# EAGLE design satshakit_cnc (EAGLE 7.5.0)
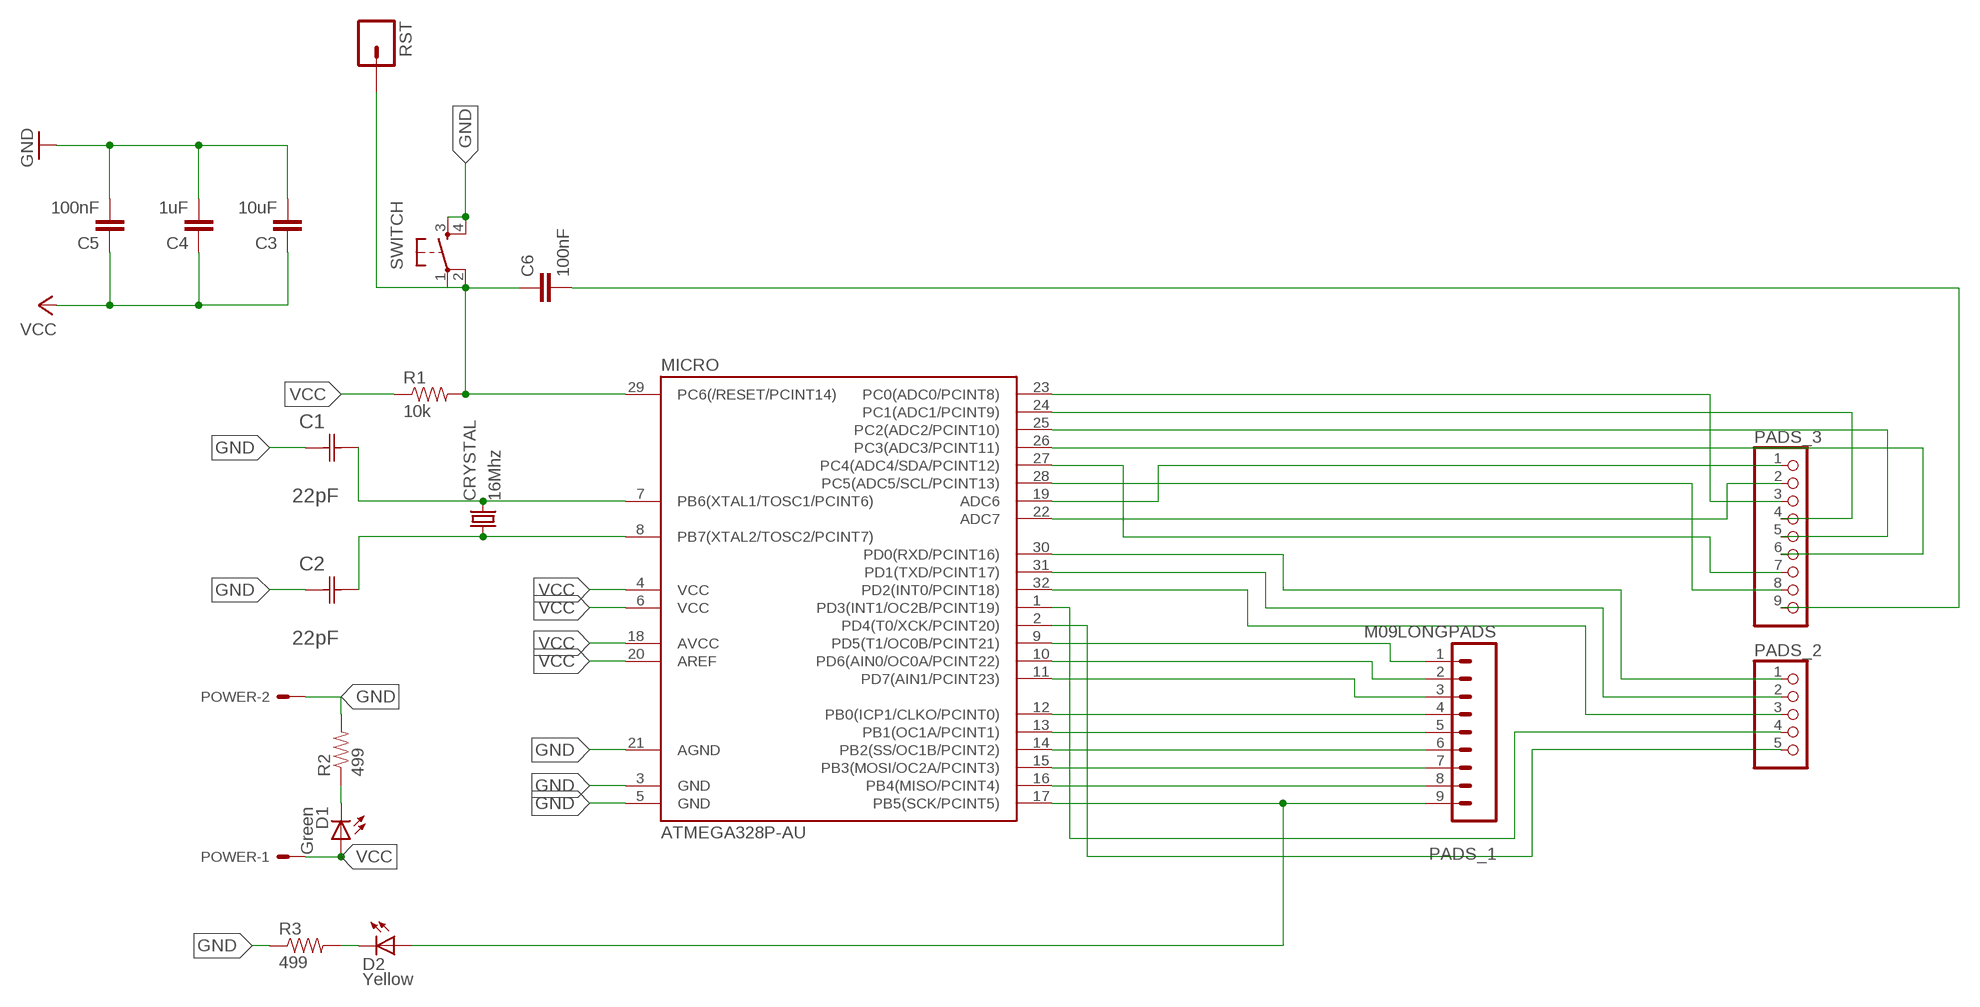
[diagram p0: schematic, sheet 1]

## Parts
C1  22pF  0612ZC225MAT2A  [CAPC3216X178N]
C2  22pF  0612ZC225MAT2A  [CAPC3216X178N]
C3  10uF  CAP1206  [1206]
C4  1uF  CAP1206  [1206]
C5  100nF  CAP1206  [1206]
C6  100nF  CAP1206  [1206]
CRYSTAL  16Mhz  CSM-7X-DU  [CSM-7X-DU]
D1  Green  LED1206  [1206]
D2  Yellow  LED1206  [1206]
MICRO  ATMEGA328P-AU  ATMEGA48/88/168-AU  [TQFP32-08]
PADS_1  M09LONGPADS  [1X09_LONGPADS]
PADS_2  PINHD-1X5  [1X05]
PADS_3  PINHD-1X9  [1X09]
POWER  22-23-2021  [22-23-2021]
R1  10k  RESISTOR1206  [1206]
R2  499  RESISTOR1206  [1206]
R3  499  RESISTOR1206  [1206]
RST  M01PTH  [1X01]
SWITCH  6MM_SWITCH6MM_SWITCH  [6MM_SWITCH]

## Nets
GND: C1.1(C1) C2.1(C1) C3.2 C4.2 C5.2 MICRO.3(GND) MICRO.5(GND) MICRO.21(AGND) POWER.2 R2.2 R3.1 SWITCH.3(S) SWITCH.4(S1)
N$1: MICRO.9(PD5(T1/OC0B/PCINT21)) PADS_1.1
N$2: C1.2(C2) CRYSTAL.2 MICRO.7(PB6(XTAL1/TOSC1/PCINT6))
N$3: C6.2 PADS_3.9
N$4: MICRO.10(PD6(AIN0/OC0A/PCINT22)) PADS_1.2
N$5: MICRO.11(PD7(AIN1/PCINT23)) PADS_1.3
N$6: MICRO.12(PB0(ICP1/CLKO/PCINT0)) PADS_1.4
N$7: MICRO.13(PB1(OC1A/PCINT1)) PADS_1.5
N$8: MICRO.14(PB2(SS/OC1B/PCINT2)) PADS_1.6
N$9: C2.2(C2) CRYSTAL.1 MICRO.8(PB7(XTAL2/TOSC2/PCINT7))
N$10: MICRO.15(PB3(MOSI/OC2A/PCINT3)) PADS_1.7
N$11: MICRO.16(PB4(MISO/PCINT4)) PADS_1.8
N$12: D2.1(A) MICRO.17(PB5(SCK/PCINT5)) PADS_1.9
N$13: MICRO.19(ADC6) PADS_3.1
N$14: MICRO.22(ADC7) PADS_3.2
N$15: MICRO.23(PC0(ADC0/PCINT8)) PADS_3.3
N$16: MICRO.24(PC1(ADC1/PCINT9)) PADS_3.4
N$17: MICRO.25(PC2(ADC2/PCINT10)) PADS_3.5
N$18: MICRO.26(PC3(ADC3/PCINT11)) PADS_3.6
N$19: MICRO.27(PC4(ADC4/SDA/PCINT12)) PADS_3.7
N$20: MICRO.30(PD0(RXD/PCINT16)) PADS_2.1
N$21: MICRO.31(PD1(TXD/PCINT17)) PADS_2.2
N$22: MICRO.32(PD2(INT0/PCINT18)) PADS_2.3
N$23: MICRO.1(PD3(INT1/OC2B/PCINT19)) PADS_2.4
N$24: MICRO.2(PD4(T0/XCK/PCINT20)) PADS_2.5
N$25: MICRO.28(PC5(ADC5/SCL/PCINT13)) PADS_3.8
N$26: D1.2(C) R2.1
N$27: D2.2(C) R3.2
N$28: C6.1 MICRO.29(PC6(/RESET/PCINT14)) R1.2 RST.1 SWITCH.1(P) SWITCH.2(P1)
VCC: C3.1 C4.1 C5.1 D1.1(A) MICRO.4(VCC) MICRO.6(VCC) MICRO.18(AVCC) MICRO.20(AREF) POWER.1 R1.1

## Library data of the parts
C1 C2 = AVX_By_element14_Batch_1:0612ZC225MAT2A: Capacitor 1206; MPN: 0612ZC225MAT2A; OC_FARNELL: -; OC_NEWARK: 12N3209; SUPPLIER: AVX; TOLERANCE: ±20%; VALUE: 2.2µF; VOLTAGERATING: 10V
C3-C6 = 01_SparkFun:CAP: Capacitor
CRYSTAL = 01_FAB_Hello:CSM-7X-DU: SMD CRYSTAL; OC_FARNELL: unknown; OC_NEWARK: unknown
D1 D2 = 01_FAB_Hello:LED
MICRO = atmega8:ATMEGA48/88/168
PADS_1 = 01_SparkFun:M09: Header 9 Standard 9-pin 0.1" header. Use with straight break away headers (SKU : PRT-00116), right angle break away headers (PRT-00553), swiss pins (PRT-00743), machine pins (PRT-00117), and female headers (PRT-00115).
PADS_2 = pinhead:PINHD-1X5: PIN HEADER
PADS_3 = pinhead:PINHD-1X9: PIN HEADER
POWER = con-molex:22-23-2021: .100" (2.54mm) Center Header - 2 Pin; MF: MOLEX; MPN: 22-23-2021; OC_FARNELL: 1462926; OC_NEWARK: 25C3832
R1-R3 = 01_SparkFun:RESISTOR: Resistor
RST = 01_SparkFun:M01: Header 1
SWITCH = 01_FAB_Hello:6MM_SWITCH: OMRON SWITCH

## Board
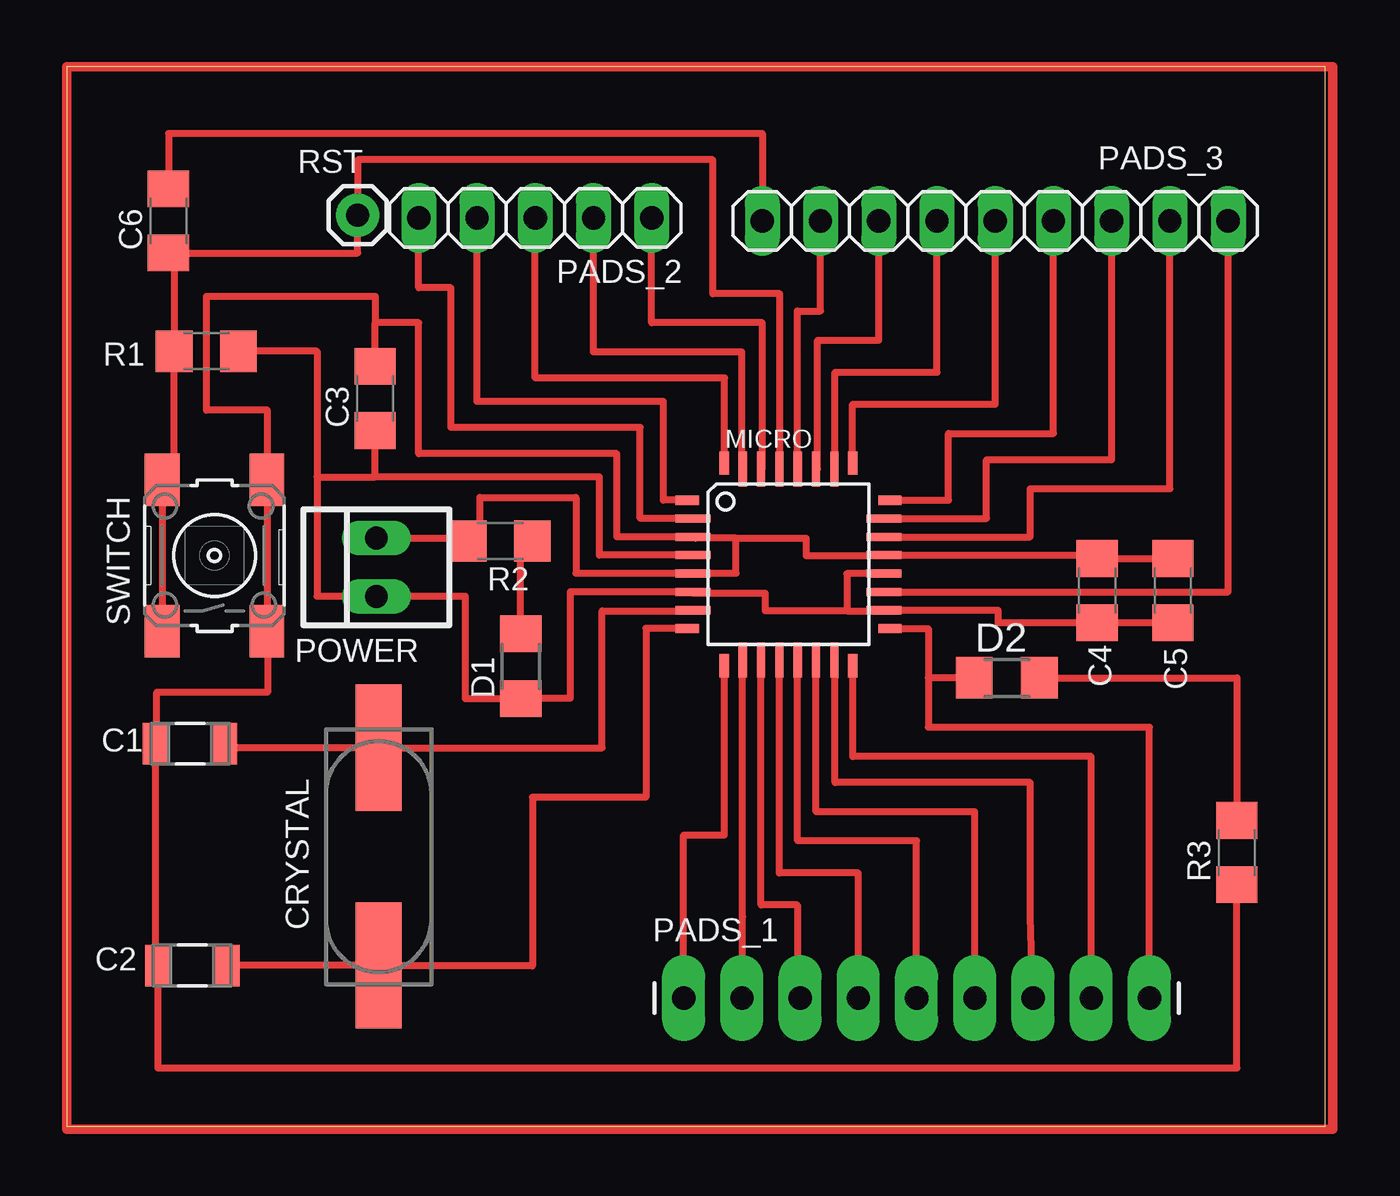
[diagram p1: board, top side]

Size 54.91 x 46.22 mm. Coordinates in mm from the lower left corner, seen from the top.
Outline: 0,0 54.91,0 54.91,46.22 0,46.22 0,0
Copper layers (1*16): Top 0.035mm / dielectric 1.5mm / Bottom 0.035mm
Design rules "default": minimum track width 10mil, minimum drill 24mil, track to track 8mil, track to pad 8mil, pad to pad 8mil, via to via 8mil, smd to smd 8mil, copper to edge 40mil, drill to drill 8mil, minimum pad ring 10mil, minimum via ring 8mil, stop-mask expansion 4mil, vias tented up to drill 0mil, thermal gap 10mil

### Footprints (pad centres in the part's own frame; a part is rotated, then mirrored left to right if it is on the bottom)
CAPC3216X178N = smd 1.118 x 1.803: 1 -1.499,0; 2 1.499,0
1206 = smd 1.6 x 1.8: 1 -1.4,0; 2 1.4,0
CSM-7X-DU = smd 5.5 x 2: 1 -4.75,0; 2 4.75,0
1206' = smd 1.6 x 1.803: 1 -1.422,0; 2 1.422,0
TQFP32-08 = smd 1.016 x 0.406: 1 -4.42,2.8; 8 -4.42,-2.8; 17 4.42,-2.8; 24 4.42,2.8 | smd 1.524 x 0.356: 2 -4.166,2; 3 -4.166,1.2; 4 -4.166,0.4; 5 -4.166,-0.4; 6 -4.166,-1.2; 7 -4.166,-2; 18 4.166,-2; 19 4.166,-1.2; 20 4.166,-0.4; 21 4.166,0.4; 22 4.166,1.2; 23 4.166,2 | smd 0.406 x 1.016: 9 -2.8,-4.42; 16 2.8,-4.42; 25 2.8,4.42; 32 -2.8,4.42 | smd 0.356 x 1.524: 10 -2,-4.166; 11 -1.2,-4.166; 12 -0.4,-4.166; 13 0.4,-4.166; 14 1.2,-4.166; 15 2,-4.166; 26 2,4.166; 27 1.2,4.166; 28 0.4,4.166; 29 -0.4,4.166; 30 -1.2,4.166; 31 -2,4.166
1X09_LONGPADS = drill 1.016 pad 1.88 long: 1 0,0; 2 2.54,0; 3 5.08,0; 4 7.62,0; 5 10.16,0; 6 12.7,0; 7 15.24,0; 8 17.78,0; 9 20.32,0
1X05 = drill 1.016 long: 1 -5.08,0; 2 -2.54,0; 3 0,0; 4 2.54,0; 5 5.08,0
1X09 = drill 1.016 long: 1 -10.16,0; 2 -7.62,0; 3 -5.08,0; 4 -2.54,0; 5 0,0; 6 2.54,0; 7 5.08,0; 8 7.62,0; 9 10.16,0
22-23-2021 = drill 1 long: 1 -1.27,0; 2 1.27,0
1X01 = drill 1.016 pad 1.88: 1 0,0
6MM_SWITCH = smd 2.286 x 1.524: 1 -3.302,2.286; 2 3.302,2.286; 3 -3.302,-2.286; 4 3.302,-2.286

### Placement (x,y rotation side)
C1  5.38,16.69 0 top
C2  5.49,7.01 0 top
C3  13.46,31.75 90 top
C4  44.96,23.37 90 top
C5  48.26,23.37 90 top
C6  4.45,39.5 90 top
CRYSTAL  13.61,11.76 90 top
D1  Green  [1206']  19.81,20.07 90 top
D2  Yellow  [1206']  41.02,19.56 0 top
MICRO  31.5,24.51 0 top
PADS_1  26.92,5.59 0 top
PADS_2  20.45,39.62 180 top
PADS_3  40.51,39.5 180 top
POWER  13.51,24.38 90 top
R1  6.1,33.81 180 top
R2  18.92,25.53 180 top
R3  51.05,11.94 90 top
RST  12.7,39.75 0 top
SWITCH  6.45,24.89 90 top

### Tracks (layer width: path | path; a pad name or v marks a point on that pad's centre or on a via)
GND
  Top 0.254: 27.36,25.68 MICRO.3 27.46,25.65 | 27.94,24.13 28.19,24.13 | 35.66,24.89 MICRO.21
  Top 0.305: MICRO.5 | MICRO.21 44.96,24.91 C4.2 C5.2 | C1.1 3.89,7.01 C2.1 3.99,2.54 51.05,2.54 R3.1 | C1.1 3.81,16.69 | 27.33,24.13 22.23,24.13 22.23,27.43 18.03,27.43 18.03,25.4 R2.2 18.03,25.65 POWER.2 | 27.33,24.13 MICRO.5 | C1.1 3.94,16.69 3.94,18.92 8.76,18.92 8.76,21.59 | 27.94,24.13 MICRO.5 | MICRO.3 24,25.71 24,29.34 15.37,29.34 15.37,35.05 13.46,35.05 | C3.2 13.46,35.05 | SWITCH.3 8.76,21.59 | 8.76,21.59 8.76,27.56 8.74,27.56 SWITCH.4 8.76,28.19 8.76,31.24 6.1,31.24 6.1,36.2 13.46,36.2 13.46,35.05 | 27.33,24.13 29.21,24.13 29.21,25.65 | 29.21,25.65 27.46,25.65 | 29.21,25.65 32.26,25.65 32.26,24.89 35.66,24.89
N$1
  Top 0.305: PADS_1.1 26.92,12.7 28.7,12.7 MICRO.9
N$2
  Top 0.305: 6.88,16.51 C1.2 6.88,16.51 | MICRO.7 27.33,22.48 23.37,22.48 23.37,16.51 CRYSTAL.2 6.88,16.51
N$3
  Top 0.305: PADS_3.9 30.35,43.31 4.45,43.31 C6.2
N$4
  Top 0.305: PADS_1.2 29.5,9.14 MICRO.10
N$5
  Top 0.305: MICRO.11 30.3,9.65 31.88,9.65 31.88,6.22 32,6.22 PADS_1.3
N$6
  Top 0.305: 31.11,20.35 MICRO.12 31.1,11.05 34.54,11.05 PADS_1.4
N$7
  Top 0.305: PADS_1.5 37.08,12.45 31.9,12.45 MICRO.13
N$8
  Top 0.305: PADS_1.6 39.62,13.72 32.7,13.72 MICRO.14
N$9
  Top 0.305: 6.99,6.99 C2.2 | MICRO.8 25.27,21.72 25.27,14.35 20.32,14.35 20.32,6.99 13.61,6.99 CRYSTAL.1 C2.2 | C2.2
N$10
  Top 0.305: PADS_1.7 42.04,9.14 42.04,14.99 33.53,14.99 33.53,19.56 MICRO.15
N$11
  Top 0.305: MICRO.16 34.3,16.13 44.7,16.13 PADS_1.8
N$12
  Top 0.305: PADS_1.9 47.24,17.4 37.59,17.4 37.59,19.56 | D2.1 37.59,19.56 | MICRO.17 37.59,21.71 37.59,19.56
N$13
  Top 0.305: MICRO.19 50.67,23.31 PADS_3.1
N$14
  Top 0.305: MICRO.22 42.04,25.71 42.04,27.81 48.13,27.81 PADS_3.2
N$15
  Top 0.305: MICRO.23 40.13,26.51 40.13,29.08 45.59,29.08 PADS_3.3
N$16
  Top 0.305: MICRO.24 38.48,27.31 38.48,30.23 43.05,30.23 PADS_3.4
N$17
  Top 0.305: MICRO.25 34.29,31.5 40.51,31.5 PADS_3.5
N$18
  Top 0.305: MICRO.26 33.53,28.68 33.53,32.89 37.97,32.89 PADS_3.6
N$19
  Top 0.305: MICRO.27 32.77,28.68 32.77,34.29 35.43,34.29 PADS_3.7
N$20
  Top 0.305: MICRO.30 30.35,28.68 30.35,35.05 25.53,35.05 PADS_2.1
N$21
  Top 0.305: MICRO.31 29.46,28.68 29.46,33.78 22.99,33.78 PADS_2.2
N$22
  Top 0.305: MICRO.32 28.7,32.64 20.45,32.64 PADS_2.3
N$23
  Top 0.305: MICRO.1 26.04,27.31 26.04,31.62 17.91,31.62 PADS_2.4
N$24
  Top 0.305: MICRO.2 25.02,26.51 25.02,30.48 16.76,30.48 16.76,36.58 15.37,36.58 PADS_2.5
N$25
  Top 0.305: MICRO.28 31.88,28.68 31.88,35.56 32.89,35.56 PADS_3.8
N$26
  Top 0.305: 20.7,25.27 R2.1 20.32,25.15 19.81,25.15 D1.2
N$27
  Top 0.305: D2.2 51.05,19.56 R3.2
N$28
  Top 0.305: MICRO.29 31.11,28.68 31.11,36.32 28.19,36.32 28.19,42.16 12.7,42.16 RST.1 12.7,38.1 4.7,38.1 | R1.2 4.44,33.81 | R1.2 4.7,28.19 SWITCH.2 SWITCH.1 | C6.1 4.7,38.1 | 4.7,38.1 R1.2
N$30
  Top 0.406: 0,-0.13 55.24,-0.13 55.24,46.23 0,46.23 0,-0.13
VCC
  Top 0.254: 35.66,22.48 MICRO.18 | 27.33,23.24 MICRO.6
  Top 0.305: MICRO.18 40.64,22.51 40.64,21.97 C4.1 C5.1 | MICRO.4 23.24,24.91 23.24,28.32 13.46,28.32 | 10.92,28.32 10.92,33.81 R1.1 | 10.92,28.32 10.92,23.11 POWER.1 17.4,23.11 17.4,18.64 D1.1 19.81,18.67 21.97,18.67 21.97,23.31 MICRO.6 28.02,23.32 | 10.92,28.32 13.46,28.32 | 13.46,28.32 C3.1 13.84,30.35 13.84,30.1 | MICRO.20 34.04,24.11 34.04,22.48 | 34.04,22.48 35.66,22.48 | 34.04,22.48 30.48,22.48 30.48,23.24 27.33,23.24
